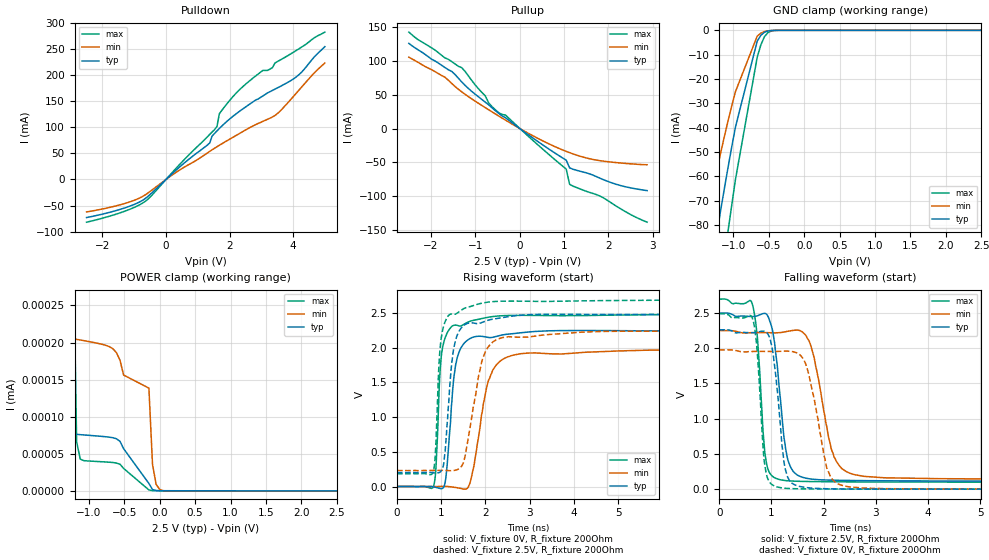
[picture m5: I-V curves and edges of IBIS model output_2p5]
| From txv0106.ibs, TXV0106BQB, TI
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|   io_2p5 Model
[Model]   output_2p5
Model_type   I/O
Polarity   Non-Inverting
Enable   Active-High
Vinl = 0.75
Vinh = 1.75
Vmeas = 1.25
Vref = 0
Cref = 2pF
Rref = 100000
|   typ   min   max
C_comp   1.540pF   1.379pF   1.78pF
| Where Nom  PVT is Nominal Process, 2.5V, 27C
|   Fast PVT is Strong Process,  2.70V, -40C
|   Slow PVT is Weak Process,   2.25, 125C
[Voltage Range]   2.5   2.25   2.75
|Junction Temperature
[Temperature Range]   27   125   -40
[Pullup Reference]   2.5   2.25   2.70
[Pulldown Reference]   0   0   0
[Power Clamp Reference]   2.5   2.25   2.70
[GND Clamp Reference]   0   0   0
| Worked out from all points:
|   slope of the pulldown table from 0 to 0.375 V, typ, clamps not added: 17.8 ohm
|   slope of the pullup table from 0 to 0.375 V, typ, clamps not added: 21.2 ohm
|   GND clamp passes 1 mA (typ) near -0.57 V on its own axis
|   POWER clamp passes 1 mA (typ) near -2.11 V on its own axis
|   falling waveform, V_fixture 2.5V, R_fixture 200Ohm: 20-80 % time 201ps typ, 325ps min, 134ps max; typ from 2.5 V to 0.112 V
|   rising waveform, V_fixture 0V, R_fixture 200Ohm: 20-80 % time 196ps typ, 344ps min, 132ps max; typ from 0 V to 2.26 V
|   rising waveform, V_fixture 2.5V, R_fixture 200Ohm: 20-80 % time 193ps typ, 346ps min, 131ps max; typ from 0.201 V to 2.5 V
|   falling waveform, V_fixture 0V, R_fixture 200Ohm: 20-80 % time 180ps typ, 304ps min, 127ps max; typ from 2.26 V to 0 V
[Pulldown]
|Voltage   I(typ)   I(min)   I(max)
-2.5V     -72.93mA   -62.18mA   -81.84mA
-1.284V   -54.21mA   -45.71mA   -60.47mA
-600mV    -34mA      -27.28mA   -39.41mA
1.376V    70.01mA    53.84mA    86.42mA
1.528V    88.23mA    59.87mA    95.56mA
1.604V    93.06mA    62.78mA    101.5mA
1.68V     97.76mA    65.62mA    126.1mA
2.364V    132.9mA    89.94mA    174.9mA
3.352V    170.8mA    119.9mA    214.5mA
3.504V    175.5mA    126.2mA    225.9mA
4.188V    201.1mA    171.5mA    250.6mA
5V        254.5mA    223.2mA    282.5mA
[GND Clamp]
|Voltage   I(typ)   I(min)   I(max)
-2.092V   -248.6mA   -191.1mA   -306.3mA
-1.429V   -119.5mA   -85.39mA   -158.7mA
-1.378V   -109.9mA   -77.92mA   -147.5mA
-1.225V   -82.07mA   -56.47mA   -114.1mA
-1.174V   -73.11mA   -49.69mA   -103.2mA
-1.072V   -55.84mA   -36.85mA   -81.8mA
-970mV    -39.69mA   -25.16mA   -61.25mA
-664mV    -4.475mA   -2.4mA     -11.11mA
-613mV    -2.08mA    -1.169mA   -6.039mA
-511mV    -257.4uA   -192.5uA   -888.4uA
-409mV    -17.82uA   -20.92uA   -50.46uA
2.5V      0A         0A         0A
[Pullup]
|Voltage   I(typ)   I(min)   I(max)
-2.5V     125.2mA    104.9mA    141.8mA
-1.688V   89.75mA    75.53mA    103.9mA
-1.536V   84.13mA    66.42mA    98.53mA
-1.308V   68.5mA     53.93mA    89.46mA
-776mV    38.7mA     30.64mA    47.86mA
-624mV    30.31mA    24.43mA    32.05mA
-472mV    22.25mA    18.28mA    22.98mA
-320mV    15.75mA    12.27mA    19.67mA
1.048V    -46.59mA   -33.66mA   -59.73mA
1.124V    -57.9mA    -35.55mA   -82.05mA
1.808V    -73.08mA   -47.32mA   -99.3mA
2.872V    -91.35mA   -53.32mA   -137.8mA
[POWER Clamp]
|Voltage  I(typ)   I(min)   I(max)
-2.447V   8.266mA    1.188mA    23.04mA
-1.631V   89.36uA    410.3nA    361.9uA
-1.427V   625.7nA    209.2nA    115.9uA
-1.325V   88.21nA    207nA      22.38uA
-1.223V   76.84nA    205.2nA    354.5nA
-1.172V   76.27nA    204.3nA    66.24nA
-1.121V   75.86nA    203.5nA    42.95nA
-560mV    66.92nA    176.2nA    36nA
-152mV    10.06nA    138.6nA    1.335nA
-101mV    1.901nA    35.68nA    364.7pA
1mV       333.1pA    1.981nA    228.7pA
2.5V      0A         0A         0A
[Ramp]
R_load = 200
|   typ   min   max
dV/dt_r   1.357/0.194n   1.186/0.338n   1.494/0.131n
dV/dt_f   1.433/0.200n   1.270/0.330n   1.559/0.135n
[Falling Waveform]
V_fixture = 2.5V
V_fixture_min = 2.25V
V_fixture_max = 2.70V
R_fixture = 200Ohm
C_fixture = 0F
|   Time   V(typ)   V(min)   V(max)
0s        2.499V     2.25V      2.697V
630ps     2.45V      2.222V     2.638V
730ps     2.46V      2.223V     2.167V
930ps     2.457V     2.221V     290.6mV
1.06ns    2.082V     2.219V     162.5mV
1.3ns     461.5mV    2.24V      119.7mV
1.67ns    154.9mV    2.17V      109.2mV
2.35ns    125mV      291.1mV    104mV
4.24ns    115.7mV    148.7mV    100.5mV
200ns     111.6mV    133.5mV    99.26mV
[Rising Waveform]
|Gnd
V_fixture = 0V
V_fixture_min = 0V
V_fixture_max = 0V
R_fixture = 200Ohm
C_fixture = 0F
|   Time   V(typ)   V(min)   V(max)
0s        10.67uV    11.98uV    10.56uV
830ps     -5.229mV   -161.4uV   7.448mV
880ps     -12.37mV   -39.02uV   257.9mV
980ps     -29.09mV   1.431mV    1.714V
1.06ns    -5.242mV   1.989mV    2.081V
1.32ns    1.728V     -13.26mV   2.323V
1.59ns    2.104V     -26.83mV   2.361V
2.07ns    2.144V     1.533V     2.436V
2.62ns    2.2V       1.89V      2.462V
200ns     2.262V     1.977V     2.489V
[Rising Waveform]
V_fixture = 2.5V
V_fixture_min = 2.25V
V_fixture_max = 2.70V
R_fixture = 200Ohm
C_fixture = 0F
|   Time   V(typ)   V(min)   V(max)
0s        200.8mV    230mV      184.1mV
810ps     198.5mV    231.5mV    196.3mV
860ps     195.2mV    231.7mV    391mV
950ps     200.1mV    232.8mV    1.76V
1.02ns    248.7mV    233.4mV    2.215V
1.26ns    1.895V     228.8mV    2.483V
1.45ns    2.28V      283mV      2.538V
1.93ns    2.363V     1.828V     2.639V
2.38ns    2.43V      2.143V     2.667V
200ns     2.499V     2.25V      2.697V
[Falling Waveform]
V_fixture = 0V
V_fixture_min = 0V
V_fixture_max = 0V
R_fixture = 200Ohm
C_fixture = 0F
|   Time   V(typ)   V(min)   V(max)
0s        2.262V     1.977V     2.489V
630ps     2.22V      1.954V     2.439V
720ps     2.226V     1.955V     2.016V
860ps     2.241V     1.955V     412.3mV
950ps     2.179V     1.954V     115.6mV
1.27ns    272.6mV    1.959V     12.57mV
1.57ns    34.89mV    1.889V     4.497mV
2.13ns    5.192mV    178.2mV    1.691mV
3.21ns    1.199mV    6.972mV    620.2uV
200ns     -325.9nV   -258.8nV   -137.8nV
